(* 	
	Program Name: 	ACS_CMD_CLEAR_START_MOTION
	Purpose:		Copy Enable Command to ACS Drive Output Command Register
	When Executed:	Enables the drive, does not interrupt move in progress
*)
PROGRAM ACS_CMD_CLEAR_START_MOTION
VAR_IN_OUT
	Axis:ACS_DRIVE_TYPE;
END_VAR
VAR
	_command:	USINT	:= ACS_COMMANDS.CLEAR_START_MOTION;
END_VAR

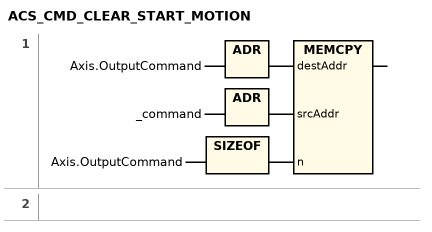
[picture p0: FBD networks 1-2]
// NETWORK 1
MEMCPY(destAddr := ADR(Axis.OutputCommand), srcAddr := ADR(_command), n := SIZEOF(Axis.OutputCommand));

// NETWORK 2

END_PROGRAM
